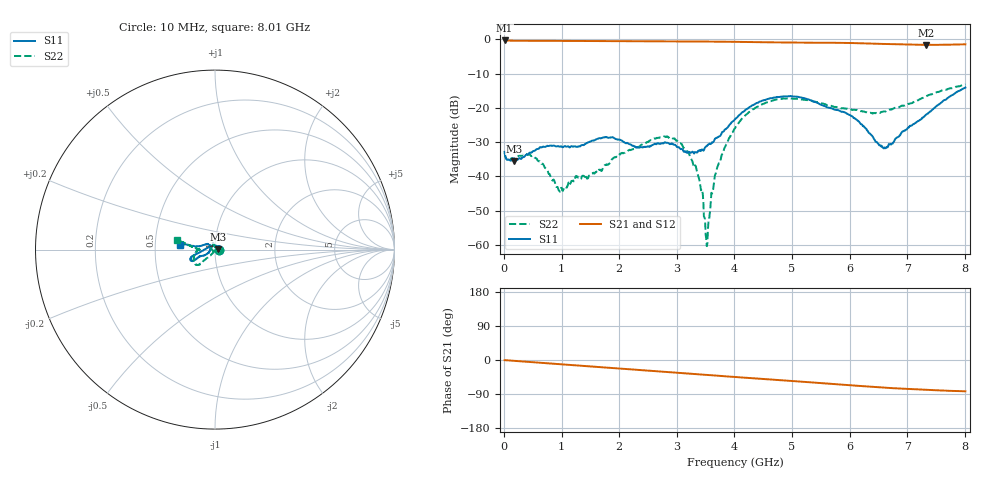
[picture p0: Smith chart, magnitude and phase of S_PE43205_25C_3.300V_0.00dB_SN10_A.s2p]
! Device ID: PE43205
! Dir: z:\David_A\43205\PE43701\25C\3p300V\0p00dB
! Serial: 10
! Insertion: A
! Impedance: 50 ohm
! Temp: 25C
! VDD: 3.300V
! Attenuation Step: 0.00dB
! IDD: 1.237241e-01mA
#  Hz  S  RI  R  50
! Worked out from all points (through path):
!   801 points, 10 MHz to 8.01 GHz, reference 50 ohm
!   highest |S21| = -0.29 dB at 10 MHz (marker M1); lowest = -1.6 dB at 7.32 GHz (marker M2)
!   group delay of S21, straight-line fit = 29.8 ps
!   lowest |S11| = -35.5 dB at 180 MHz (marker M3), VSWR 1.03, Z = 51.7 + j0.277 ohm
!   |S11| at or under -10 dB: start of sweep to end of sweep
!   |S22| runs from -60.4 to -13.1 dB; largest |S21 - S12| = 0.0061
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1e7  0.0223 -0.00497  0.9672 -0.00705  0.967 -0.00743  0.022 -0.0044
1.8e8  0.0165 0.00268  0.9586 -0.0367  0.9588 -0.0366  0.018 0.00356
5.3e8  0.0232 0.00369  0.9508 -0.1017  0.951 -0.1019  0.0176 0.00649
9.8e8  0.0259 -0.00832  0.9351 -0.1841  0.935 -0.1842  0.00559 -0.00303
1.35e9  0.0213 -0.019  0.9161 -0.2507  0.9161 -0.2507  -0.00278 -0.00951
1.76e9  0.03 -0.0226  0.8907 -0.3212  0.8908 -0.3213  -0.0139 -0.00449
2.32e9  0.0268 0.00154  0.8471 -0.4127  0.847 -0.4126  -0.017 0.0205
2.68e9  0.0269 0.0134  0.8138 -0.4683  0.8134 -0.4681  -0.0135 0.0341
2.97e9  0.0227 0.018  0.7841 -0.5118  0.7841 -0.5116  -0.00878 0.0337
3.23e9  0.00721 0.021  0.7551 -0.5489  0.7554 -0.5491  -0.00324 0.019
3.41e9  -0.00764 0.0221  0.7342 -0.5746  0.7342 -0.5745  0.00177 0.00686
3.49e9  -0.0147 0.0219  0.7247 -0.5862  0.7248 -0.5859  6.18e-05 0.00236
3.52e9  -0.0173 0.0215  0.7205 -0.59  0.7207 -0.59  0.000946 -0.000122
3.69e9  -0.0331 0.0157  0.6983 -0.6128  0.6984 -0.6125  -0.00515 -0.0112
4.01e9  -0.0682 -0.00562  0.6537 -0.6517  0.6538 -0.6519  -0.0337 -0.0376
4.58e9  -0.1291 -0.0378  0.5709 -0.7072  0.5706 -0.7065  -0.0882 -0.0835
5.35e9  -0.113 -0.0577  0.4597 -0.7678  0.4599 -0.7672  -0.1169 -0.0457
6.01e9  -0.0708 -0.034  0.3528 -0.8134  0.3529 -0.8144  -0.0958 -0.00132
6.55e9  -0.0271 -0.00162  0.2581 -0.8221  0.2595 -0.8217  -0.0873 0.00032
6.68e9  -0.0269 0.0122  0.2398 -0.8225  0.2399 -0.8214  -0.0942 -0.000609
7.32e9  -0.0755 0.0218  0.1646 -0.8173  0.1628 -0.8165  -0.1436 0.0246
8.01e9  -0.1963 0.028  0.1093 -0.8422  0.1065 -0.8476  -0.214 0.0537
